|   stm32f0_448_ufbga100 IBIS Model
[IBIS ver]   4.2
[File name]  stm32f0_448_ufbga100.ibs
[File Rev]   1.0
[Date]   15-5-2013
[Source] Data Created at STMicroelectronics
[Notes]   File originated from ELDO simulations.
[Disclaimer]  This information is for modeling purpose only and is
   not guaranted. The information is subject to change without
   notice.
[Copyright] Copyright 2015 STMicroelectronics Inc.
[Component] stm32f0_448_ufbga100
[Manufacturer] STMicroelectronics
[Package]
| variable   typ   min   max
R_pkg   0.0   NA   NA
L_pkg   0.0H   NA   NA
C_pkg   0.0F   NA   NA
[Pin] signal_name  model_name   R_pin   L_pin   C_pin
B2   PE2   io8p_sudq_ft   0.132430474   7.03E-09   1.35E-13
A1   PE3   io8p_sudq_ft   0.133347678   6.77E-09   1.95E-14
B1   PE4   io8p_sudq_ft   0.12897311   6.49E-09   1.04E-14
C2   PE5   io8p_sudq_ft   0.125344562   6.21E-09   5.24E-15
D2   PE6   io8p_sudq_ft   0.120515446   5.99E-09   7.82E-15
E2   VBAT   POWER   0.12047071   5.95E-09   6.53E-15
C1   PC13   io8p_sudq_tc   0.117880646   5.78E-09   6.23E-15
D1   PC14   io8p_sudq_tc   0.117278614   5.65E-09   3.11E-15
E1   PC15   io8p_sudq_tc   0.11554812   5.55E-09   1.39E-15
F2   PF9   io8p_sudq_ft   0.114995632   5.43E-09   2.92E-15
G2   PF10   io8p_sudq_ft   0.112975638   5.30E-09   3.56E-15
F1   PF0   io8p_sudq_ft   0.111323436   5.23E-09   4.78E-15
G1   PF1   io8p_sudq_ft   0.109216856   5.14E-09   8.66E-15
H2   NRST   ioreset_tc_v33   0.11066442   5.18E-09   9.03E-15
H1   PC0   io8p_sudq_ft   0.110607546   5.19E-09   7.98E-15
J2   PC1   io8p_sudq_ft   0.111326184   5.25E-09   1.03E-14
J3   PC2   io8p_sudq_ft   0.11442005   5.35E-09   7.00E-15
K2   PC3   io8p_sudq_ft   0.114363236   5.45E-09   8.65E-15
J1   PF2   io8p_sudq_ft   0.117563732   5.62E-09   7.83E-15
K1   VSSA   GND   0.119904688   5.80E-09   2.29E-16
M1   VDDA   POWER   0.122311852   5.96E-09   1.05E-15
L1   PF3   io8p_sudq_ft   0.125384354   6.19E-09   8.12E-16
L2   PA0   io8p_sudq_ft   0.129702038   6.49E-09   3.82E-15
M2   PA1   io8p_sudq_ft   0.13229018   6.71E-09   6.80E-15
K3   PA2   io8p_sudq_ft   0.132955142   7.01E-09   1.67E-14
L3   PA3   io8p_sudq_ft   0.13394318   7.05E-09   1.75E-14
D3   VSS   GND   0.13495773   6.80E-09   1.27E-14
H3   VDD   POWER   0.130511464   6.53E-09   9.83E-15
M3   PA4   io8p_sudq_ft   0.1253867   6.24E-09   6.07E-15
K4   PA5   io8p_sudq_ft   0.124988978   6.11E-09   5.77E-16
L4   PA6   io8p_sudq_ft   0.121784338   5.89E-09   1.52E-15
M4   PA7   io8p_sudq_ft   0.119149388   5.72E-09   5.44E-15
K5   PC4   io8p_sudq_ft   0.116374808   5.56E-09   4.10E-15
L5   PC5   io8p_sudq_ft   0.113278606   5.41E-09   3.69E-15
M5   PB0   io8p_sudq_ft   0.112726654   5.36E-09   3.90E-15
M6   PB1   io8p_sudq_ft   0.112271006   5.27E-09   1.66E-15
L6   PB2   io8p_sudq_ft   0.111816114   5.24E-09   7.92E-15
M7   PE7   io8p_sudq_ft   0.110998514   5.18E-09   9.90E-15
L7   PE8   io8p_sudq_ft   0.114588522   5.30E-09   7.91E-15
M8   PE9   io8p_sudq_ft   0.114461118   5.33E-09   7.94E-15
L8   PE10   io8p_sudq_ft   0.11535023   5.42E-09   4.18E-15
M9   PE11   io8p_sudq_ft   0.116979452   5.53E-09   6.06E-15
L9   PE12   io8p_sudq_ft   0.120184998   5.70E-09   5.12E-15
M10   PE13   io8p_sudq_ft   0.12258702   5.87E-09   4.74E-15
M11   PE14   io8p_sudq_ft   0.126303358   6.07E-09   1.16E-14
M12   PE15   io8p_sudq_ft   0.129714658   6.28E-09   9.91E-15
L10   PB10   io8p_sudq_i2cin_lv_ft   0.133373154   6.51E-09   5.08E-15
L11   PB11   io8p_sudq_i2cin_lv_ft   0.137888146   6.86E-09   5.47E-15
F12   VSS   GND   0.131554082   6.80E-09   4.18E-15
G12   VDD   POWER   0.132347744   7.04E-09   1.19E-14
L12   PB12   io8p_sudq_ft   0.131767814   7.01E-09   1.62E-14
K12   PB13   io8p_sudq_ft   0.131784366   6.75E-09   2.15E-15
K11   PB14   io8p_sudq_ft   0.129150704   6.48E-09   9.18E-15
K10   PB15   io8p_sudq_ft   0.12519135   6.20E-09   5.66E-15
K9   PD8   io8p_sudq_ft   0.121530258   5.99E-09   3.69E-15
K8   PD9   io8p_sudq_ft   0.11887369   5.81E-09   7.43E-15
J12   PD10   io8p_sudq_ft   0.11586992   5.64E-09   1.06E-14
J11   PD11   io8p_sudq_ft   0.113225758   5.47E-09   5.76E-15
J10   PD12   io8p_sudq_ft   0.111781608   5.35E-09   6.53E-15
H12   PD13   io8p_sudq_ft   0.110712606   5.28E-09   1.14E-14
H11   PD14   io8p_sudq_ft   0.110051596   5.20E-09   1.32E-14
H10   PD15   io8p_sudq_ft   0.10995365   5.18E-09   1.46E-14
E12   PC6   io8p_sudq_ft   0.1097803   5.15E-09   7.25E-15
E11   PC7   io8p_sudq_ft   0.112445854   5.26E-09   3.59E-16
E10   PC8   io8p_sudq_ft   0.113595842   5.33E-09   6.58E-16
D12   PC9   io8p_sudq_ft   0.115707136   5.47E-09   5.09E-16
D11   PA8   io8p_sudq_ft   0.116952062   5.60E-09   5.83E-16
D10   PA9   io8p_sudq_ft   0.11904328   5.76E-09   5.46E-16
C12   PA10   io8p_sudq_ft   0.120673854   5.88E-09   1.39E-14
B12   PA11   io8p_sudq_ft   0.124658692   6.11E-09   2.50E-14
A12   PA12   io8p_sudq_ft   0.124406978   6.16E-09   3.99E-14
A11   PA13   io8p_sudq_ft   0.130155984   6.40E-09   3.02E-13
C11   PF6   io8p_sudq_i2cin_lv_ft   0.135109698   6.82E-09   1.55E-13
F11   VSS   GND   0.139401952   7.08E-09   1.55E-13
G11   VDDIO2  POWER   0.133554014   7.06E-09   3.90E-14
A10   PA14   io8p_sudq_ft   0.135294596   7.10E-09   1.63E-14
A9   PA15   io8p_sudq_ft   0.132513704   6.84E-09   9.76E-15
B11   PC10   io8p_sudq_ft   0.133481516   6.64E-09   9.30E-15
C10   PC11   io8p_sudq_ft   0.12836612   6.34E-09   5.42E-15
B10   PC12   io8p_sudq_ft   0.124282386   6.09E-09   1.18E-15
C9   PD0   io8p_sudq_ft   0.121841172   5.92E-09   5.46E-15
B9   PD1   io8p_sudq_ft   0.118487054   5.73E-09   7.00E-15
C8   PD2   io8p_sudq_ft   0.117180194   5.57E-09   6.06E-15
B8   PD3   io8p_sudq_ft   0.11350052   5.42E-09   5.45E-15
B7   PD4   io8p_sudq_ft   0.113789098   5.34E-09   5.29E-16
A6   PD5   io8p_sudq_ft   0.110805858   5.26E-09   2.99E-15
B6   PD6   io8p_sudq_ft   0.110442376   5.25E-09   2.06E-15
A5   PD7   io8p_sudq_ft   0.111525472   5.18E-09   5.68E-15
A8   PB3   io8p_sudq_ft   0.11114441   5.22E-09   9.91E-15
A7   PB4   io8p_sudq_ft   0.113222316   5.31E-09   9.05E-15
C5   PB5   io8p_sudq_ft   0.113322882   5.40E-09   1.29E-14
B5   PB6   io8p_sudq_i2cin_lv_ft   0.1158486   5.52E-09   1.26E-14
B4   PB7   io8p_sudq_i2cin_lv_ft   0.117577758   5.67E-09   6.14E-15
A4   BOOT0   vpp_test_hv   0.1189821   5.80E-09   9.37E-15
A3   PB8   io8p_sudq_i2cin_lv_ft   0.121885942   5.96E-09   7.76E-15
B3   PB9   io8p_sudq_i2cin_lv_ft   0.126275558   6.16E-09   8.56E-15
C3   PE0   io8p_sudq_ft   0.128749356   6.37E-09   8.16E-15
A2   PE1   io8p_sudq_ft   0.13328845   6.70E-09   1.03E-15
|D3   VSS   GND   0.13223018   6.84E-09   4.41E-15
C4   VDD   POWER   0.132277204   7.05E-09   1.71E-14
[Model Selector] io8p_sudq_ft
io8p01_sudq_ft_pd_lv  "SPEED01 2P0V, PD=40kOhm"
io8p01_sudq_ft_pu_lv  "SPEED01 2P0V, PU=40kOhm"
io8p01_sudq_ft_lv  "SPEED01 2P0V"
io8p10_sudq_ft_pd_lv  "SPEED10 2P0V, PD=40kOhm"
io8p10_sudq_ft_pu_lv  "SPEED10 2P0V, PU=40kOhm"
io8p10_sudq_ft_lv  "SPEED10 2P0V"
io8p11_sudq_ft_pd_lv  "SPEED11 2P0V, PD=40kOhm"
io8p11_sudq_ft_pu_lv  "SPEED11 2P0V, PU=40kOhm"
io8p11_sudq_ft_lv  "SPEED11 2P0V"
io8p01_sudq_ft_pd  "SPEED01, PD=40kOhm"
io8p01_sudq_ft_pu  "SPEED01, PU=40kOhm"
io8p01_sudq_ft  "SPEED01"
io8p10_sudq_ft_pd  "SPEED10, PD=40kOhm"
io8p10_sudq_ft_pu  "SPEED10, PU=40kOhm"
io8p10_sudq_ft  "SPEED10"
io8p11_sudq_ft_pd  "SPEED11, PD=40kOhm"
io8p11_sudq_ft_pu  "SPEED11, PU=40kOhm"
io8p11_sudq_ft  "SPEED11"
[Model Selector] io8p_sudq_i2cin_lv_ft
io8p01_sudq_i2cin_lv_ft_pd_lv  "SPEED01 2P0V, PD=40kOhm"
io8p01_sudq_i2cin_lv_ft_pu_lv  "SPEED01 2P0V, PU=40kOhm"
io8p01_sudq_i2cin_lv_ft_lv  "SPEED01 2P0V"
io8p10_sudq_i2cin_lv_ft_pd_lv  "SPEED10 2P0V, PD=40kOhm"
io8p10_sudq_i2cin_lv_ft_pu_lv  "SPEED10 2P0V, PU=40kOhm"
io8p10_sudq_i2cin_lv_ft_lv  "SPEED10 2P0V"
io8p11_sudq_i2cin_lv_ft_pd_lv  "SPEED11 2P0V, PD=40kOhm"
io8p11_sudq_i2cin_lv_ft_pu_lv  "SPEED11 2P0V, PU=40kOhm"
io8p11_sudq_i2cin_lv_ft_lv  "SPEED11 2P0V"
io8p01_sudq_i2cin_lv_ft_pd  "SPEED01, PD=40kOhm"
io8p01_sudq_i2cin_lv_ft_pu  "SPEED01, PU=40kOhm"
io8p01_sudq_i2cin_lv_ft  "SPEED01"
io8p10_sudq_i2cin_lv_ft_pd  "SPEED10, PD=40kOhm"
io8p10_sudq_i2cin_lv_ft_pu  "SPEED10, PU=40kOhm"
io8p10_sudq_i2cin_lv_ft  "SPEED10"
io8p11_sudq_i2cin_lv_ft_pd  "SPEED11, PD=40kOhm"
io8p11_sudq_i2cin_lv_ft_pu  "SPEED11, PU=40kOhm"
io8p11_sudq_i2cin_lv_ft  "SPEED11"
[Model Selector] io8p_sudq_tc
io8p01_sudq_tc_pd_lv  "SPEED01 2P0V, PD=40kOhm"
io8p01_sudq_tc_pu_lv  "SPEED01 2P0V, PU=40kOhm"
io8p01_sudq_tc_lv  "SPEED01 2P0V"
io8p10_sudq_tc_pd_lv  "SPEED10 2P0V, PD=40kOhm"
io8p10_sudq_tc_pu_lv  "SPEED10 2P0V, PU=40kOhm"
io8p10_sudq_tc_lv  "SPEED10 2P0V"
io8p11_sudq_tc_pd_lv  "SPEED11 2P0V, PD=40kOhm"
io8p11_sudq_tc_pu_lv  "SPEED11 2P0V, PU=40kOhm"
io8p11_sudq_tc_lv  "SPEED11 2P0V"
io8p01_sudq_tc_pd  "SPEED01, PD=40kOhm"
io8p01_sudq_tc_pu  "SPEED01, PU=40kOhm"
io8p01_sudq_tc  "SPEED01"
io8p10_sudq_tc_pd  "SPEED10, PD=40kOhm"
io8p10_sudq_tc_pu  "SPEED10, PU=40kOhm"
io8p10_sudq_tc  "SPEED10"
io8p11_sudq_tc_pd  "SPEED11, PD=40kOhm"
io8p11_sudq_tc_pu  "SPEED11, PU=40kOhm"
io8p11_sudq_tc  "SPEED11"
[Model Selector] ioreset_tc_v33
ioreset_tc_v33_pu_lv  "IORESET 2V + PU=40kOhm"
ioreset_tc_v33_nopu_lv  "IORESET 2V"
ioreset_tc_v33_pu  "IORESET + PU=40kOhm"
ioreset_tc_v33_nopu  "IORESET"
[Model Selector] vpp_test_hv
vpp_test_hv_3p3  "Input Buffer"
vpp_test_hv_2p4  "Input Buffer 2P0V"
| Models and submodels in the file (60): io8p01_sudq_ft_pd_lv (I/O), io8p01_sudq_ft_pu_lv (I/O), io8p01_sudq_ft_lv (I/O), io8p10_sudq_ft_pd_lv (I/O), io8p10_sudq_ft_pu_lv (I/O), io8p10_sudq_ft_lv (I/O), io8p11_sudq_ft_pd_lv (I/O), io8p11_sudq_ft_pu_lv (I/O), io8p11_sudq_ft_lv (I/O), io8p01_sudq_ft_pd (I/O), io8p01_sudq_ft_pu (I/O), io8p01_sudq_ft (I/O), io8p10_sudq_ft_pd (I/O), io8p10_sudq_ft_pu (I/O), io8p10_sudq_ft (I/O), io8p11_sudq_ft_pd (I/O), io8p11_sudq_ft_pu (I/O), io8p11_sudq_ft (I/O), io8p01_sudq_i2cin_lv_ft_pd_lv (I/O), io8p01_sudq_i2cin_lv_ft_pu_lv (I/O), io8p01_sudq_i2cin_lv_ft_lv (I/O), io8p10_sudq_i2cin_lv_ft_pd_lv (I/O), io8p10_sudq_i2cin_lv_ft_pu_lv (I/O), io8p10_sudq_i2cin_lv_ft_lv (I/O), io8p11_sudq_i2cin_lv_ft_pd_lv (I/O), io8p11_sudq_i2cin_lv_ft_pu_lv (I/O), io8p11_sudq_i2cin_lv_ft_lv (I/O), io8p01_sudq_i2cin_lv_ft_pd (I/O), io8p01_sudq_i2cin_lv_ft_pu (I/O), io8p01_sudq_i2cin_lv_ft (I/O), io8p10_sudq_i2cin_lv_ft_pd (I/O), io8p10_sudq_i2cin_lv_ft_pu (I/O), io8p10_sudq_i2cin_lv_ft (I/O), io8p11_sudq_i2cin_lv_ft_pd (I/O), io8p11_sudq_i2cin_lv_ft_pu (I/O), io8p11_sudq_i2cin_lv_ft (I/O), io8p01_sudq_tc_pd_lv (I/O), io8p01_sudq_tc_pu_lv (I/O), io8p01_sudq_tc_lv (I/O), io8p10_sudq_tc_pd_lv (I/O), io8p10_sudq_tc_pu_lv (I/O), io8p10_sudq_tc_lv (I/O), io8p11_sudq_tc_pd_lv (I/O), io8p11_sudq_tc_pu_lv (I/O), io8p11_sudq_tc_lv (I/O), io8p01_sudq_tc_pd (I/O), io8p01_sudq_tc_pu (I/O), io8p01_sudq_tc (I/O), io8p10_sudq_tc_pd (I/O), io8p10_sudq_tc_pu (I/O), io8p10_sudq_tc (I/O), io8p11_sudq_tc_pd (I/O), io8p11_sudq_tc_pu (I/O), io8p11_sudq_tc (I/O), ioreset_tc_v33_pu_lv (I/O_open_drain), ioreset_tc_v33_nopu_lv (I/O_open_drain), ioreset_tc_v33_pu (I/O_open_drain), ioreset_tc_v33_nopu (I/O_open_drain), vpp_test_hv_2p4 (Input), vpp_test_hv_3p3 (Input)
